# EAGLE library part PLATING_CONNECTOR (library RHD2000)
CnC Tech 10-pin right angle connector (DigiKey 1175-1628-ND)
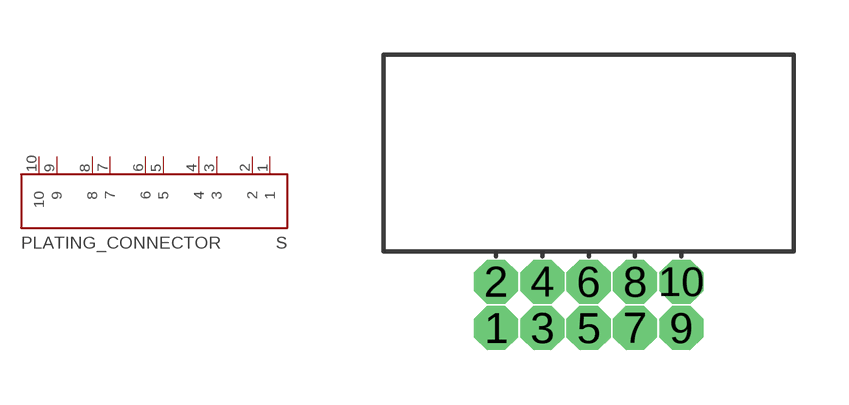
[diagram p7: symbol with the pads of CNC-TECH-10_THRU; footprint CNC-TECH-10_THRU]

Designator prefix S

## PLATING_CONNECTOR  [CNC-TECH-10_THRU]
1  1
2  2
3  3
4  4
5  5
6  6
7  7
8  8
9  9
10  10

## Footprint CNC-TECH-10_THRU (pad centres in mm)
drill 0.7 pad 1.05 octagon: 1 -2.54,-1.27; 2 -2.54,0; 3 -1.27,-1.27; 4 -1.27,0; 5 0,-1.27; 6 0,0; 7 1.27,-1.27; 8 1.27,0; 9 2.54,-1.27; 10 2.54,0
